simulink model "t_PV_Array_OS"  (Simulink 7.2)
settings: Solver=ode3  StartTime=0.0  StopTime=0.005  FixedStep=10e-6  MaxStep=1e-5  RelTol=1e-5  AbsTol=1e-5
libraries: simulink x2

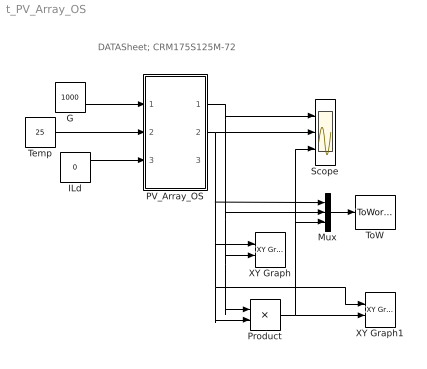
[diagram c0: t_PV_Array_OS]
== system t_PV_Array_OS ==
  note: DATASheet; CRM175S125M-72
  G : Constant  Value=1000
  ILd : Constant  Value=0
  Mux : Mux  Inputs=3
  PV_Array_OS : Subsystem  mask{Isc0=5.28, Ud0=44.5, Ki=2e-3, Kv=-0.1558, n=1.0, RS=0.7, RP=400, NC=72, NMs=1, NMp=1, C=1e-4, vC0=0, RL=10000}
      mask prompts: Isc0 "Short Circuit Current at STC Isc0/Module"; Ud0 "Open Circuit Voltage at STC Ud0/Module"; Ki "Short Circuit Current Temp Coeff. Ki/Module"; Kv "Open Circuit Voltage Temp. Coeff. Kv/Module"; n "Diode Idealty Factor n"; RS "Series Resistance Rs"; RP "Parallel Resistance RP"; NC "Number Cells"; NMs "Number Series Modules"; NMp "Number Parallel Modules"; C "Load Capacitor"; vC0 "init Cap Voltage"; RL "Load Res."
      mask help: PV_Array_OS with parameters: N_Cells/Module (NC), N_Series connected Module (NMs) and N_parallel connected Module (NMp) Input Vector u: u[0]=G u[1]=T u[2]=ILd Output Vector y: y[0]=PV.I y[1]=PV.V y[2]=C.I Parameter Vector p: p[0]=Isc0 p[1]=Ud0 p[2]=Ki p[3]=Kv p[4]=n p[5]=RS p[6]=RP p[7]=NC p[8]=NMs p[9]=NMp p[10]=C p[11]=vC0 p[12]=RL You can pause the simulation during running, change the Parameters you want and continue the Simulation
  Product : Product
  Scope : Scope  NumInputPorts=3
  Temp : Constant  Value=25
  ToW : ToWorkspace  VariableName=Y_VIP_25  SampleTime=-1  SaveFormat=Array
  XY Graph : simulink/Sinks/XY Graph  SystemSampleTime=-1  xmin=0  xmax=50  ymin=0  ymax=6  st=-1
  XY Graph1 : simulink/Sinks/XY Graph  SystemSampleTime=-1  xmin=0  xmax=50  ymin=0  ymax=200  st=-1
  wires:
  PV_Array_OS/2(PV_V) -> Scope/2, XY Graph/1, Product/2, XY Graph1/1, Mux/1
  PV_Array_OS/1(PV_I) -> Scope/1, XY Graph/2, Product/1, Mux/2
  G/1 -> PV_Array_OS/1(G)
  Temp/1 -> PV_Array_OS/2(Temp)
  ILd/1 -> PV_Array_OS/3(ILd)
  Product/1 -> XY Graph1/2, Scope/3, Mux/3
  Mux/1 -> ToW/1

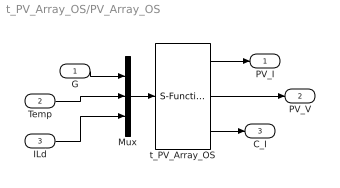
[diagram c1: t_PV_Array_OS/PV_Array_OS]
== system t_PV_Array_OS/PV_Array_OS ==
  G : Inport
  Temp : Inport  Port=2
  ILd : Inport  Port=3
  Mux : Mux  Inputs=3
  t_PV_Array_OS : S-Function  FunctionName=s_PV_Array_OS  Parameters="[Isc0  Ud0  Ki  Kv  n    RS  RP NC  NMs NMp C  vC0  RL]"  EnableBusSupport=off
  PV_I : Outport
  PV_V : Outport  Port=2
  C_I : Outport  Port=3
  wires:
  t_PV_Array_OS/3 -> C_I/1
  t_PV_Array_OS/2 -> PV_V/1
  t_PV_Array_OS/1 -> PV_I/1
  ILd/1 -> Mux/3
  Temp/1 -> Mux/2
  G/1 -> Mux/1
  Mux/1 -> t_PV_Array_OS/1
